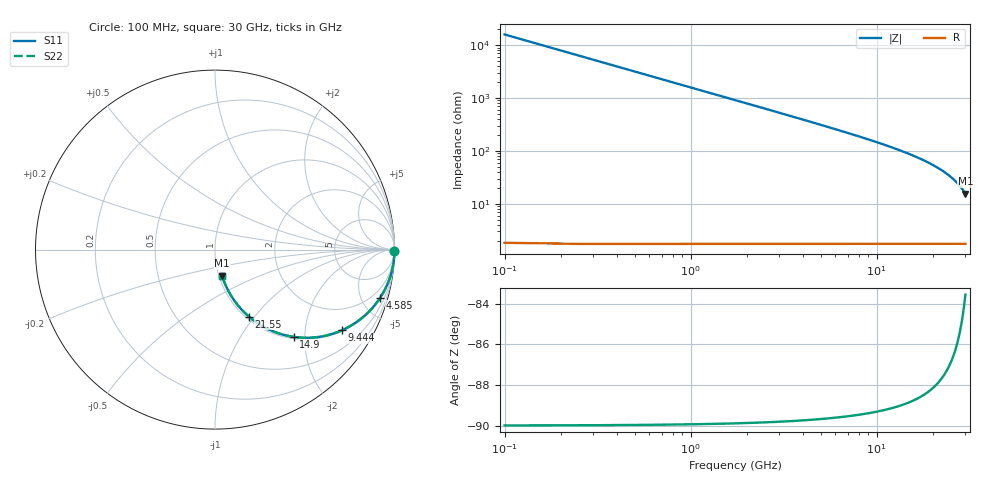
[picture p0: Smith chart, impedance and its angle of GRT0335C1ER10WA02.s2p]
!Murata Part Number: GRT0335C1ER10WA02
!These Parameters are Measured in Series Mode Connection
!Data Generated on Jun 19, 2026
!  o--ll--o
!Port1  Port2
!  o------o
!Operation Temp=25[degC], DC Bias Voltage=0[V]
!Freq. Start=100[MHz] Stop=30[GHz] 401[Steps]
# Hz S RI R 50
!Freq.(Hz) S11(Real) S11(Imag) S21(Real) S21(Imag) S12(Real) S12(Imag) S22(Real) S22(Imag)
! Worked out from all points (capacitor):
!   401 points, 100 MHz to 30 GHz, reference 50 ohm
!   read as one part in series: C = 100 fF near 249.5 MHz
!   lowest |Z| = 15.6 ohm at 30 GHz (marker M1)
!   S11 on the Smith chart (normalised r, x): 100 MHz: open; 4.585 GHz: 1.03, -6.83; 9.444 GHz: 1.03, -3.13; 14.9 GHz: 1.03, -1.76; 21.55 GHz: 1.03, -0.94; 30 GHz: 1.03, -0.31
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1e8  1 -0.00628  4.02e-05 0.00628  4.02e-05 0.00628  1 -0.00628
1.7475e8  0.9999 -0.011  0.000123 0.011  0.000123 0.011  0.9999 -0.011
3.2425e8  0.9996 -0.0204  0.000422 0.0204  0.000422 0.0204  0.9996 -0.0204
3.99e8  0.9994 -0.0251  0.000639 0.0251  0.000639 0.0251  0.9994 -0.0251
5.485e8  0.9988 -0.0344  0.00121 0.0344  0.00121 0.0344  0.9988 -0.0344
8.475e8  0.9971 -0.0531  0.00288 0.0531  0.00288 0.0531  0.9971 -0.0531
1.296e9  0.9933 -0.081  0.00672 0.081  0.00672 0.081  0.9933 -0.081
1.894e9  0.9857 -0.1176  0.0143 0.1176  0.0143 0.1176  0.9857 -0.1176
2.6415e9  0.9725 -0.1622  0.0275 0.1622  0.0275 0.1622  0.9725 -0.1622
3.5385e9  0.9512 -0.2134  0.0488 0.2134  0.0488 0.2134  0.9512 -0.2134
4.585e9  0.9198 -0.269  0.0802 0.269  0.0802 0.269  0.9198 -0.269
5.10825e9  0.9017 -0.2949  0.0983 0.2949  0.0983 0.2949  0.9017 -0.2949
7.05175e9  0.8227 -0.3779  0.1773 0.3779  0.1773 0.3779  0.8227 -0.3779
9.44375e9  0.7085 -0.4489  0.2915 0.4489  0.2915 0.4489  0.7085 -0.4489
1.01165e10  0.6747 -0.4625  0.3253 0.4625  0.3253 0.4625  0.6747 -0.4625
1.49005e10  0.4386 -0.4864  0.5614 0.4864  0.5614 0.4864  0.4386 -0.4864
1.505e10  0.4317 -0.4853  0.5683 0.4853  0.5683 0.4853  0.4317 -0.4853
2.005825e10  0.2346 -0.4079  0.7654 0.4079  0.7654 0.4079  0.2346 -0.4079
2.155325e10  0.1891 -0.3733  0.8109 0.3733  0.8109 0.3733  0.1891 -0.3733
2.50665e10  0.1061 -0.2819  0.8939 0.2819  0.8939 0.2819  0.1061 -0.2819
2.768275e10  0.0643 -0.2098  0.9357 0.2098  0.9357 0.2098  0.0643 -0.2098
3e10  0.0394 -0.1461  0.9606 0.1461  0.9606 0.1461  0.0394 -0.1461
